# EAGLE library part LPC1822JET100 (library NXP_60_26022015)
32-bit ARM Cortex-M3 MCU; up to 1 MB flash and 136 kB SRAM; Ethernet, two High-speed USB, LCD, EMC The LPC185x/3x/2x/1x are ARM Cortex-M3 based microcontrollers for embedded applications. The ARM Cortex-M3 is a next generation core that offers system enhancements such as low power consumption, enhanced debug features, and a high level of support block integration. The LPC185x/3x/2x/1x operate at CPU frequencies of up to 180 MHz. The ARM Cortex-M3 CPU incorporates a 3-stage pipeline and uses a Harvard architecture with separate local instruction and data buses as well as a third bus for peripherals. The ARM Cortex-M3 CPU also includes an internal prefetch unit that supports speculative branching. The LPC185x/3x/2x/1x include up to 1 MB of flash and 136 kB of on-chip SRAM, 16 kB of EEPROM memory, a quad SPI Flash Interface (SPIFI), a State Configurable Timer (SCT) subsystem, two High-speed USB controllers, Ethernet, LCD, an external memory controller, and multiple digital and analog peripherals. AAL Eindhoven MK
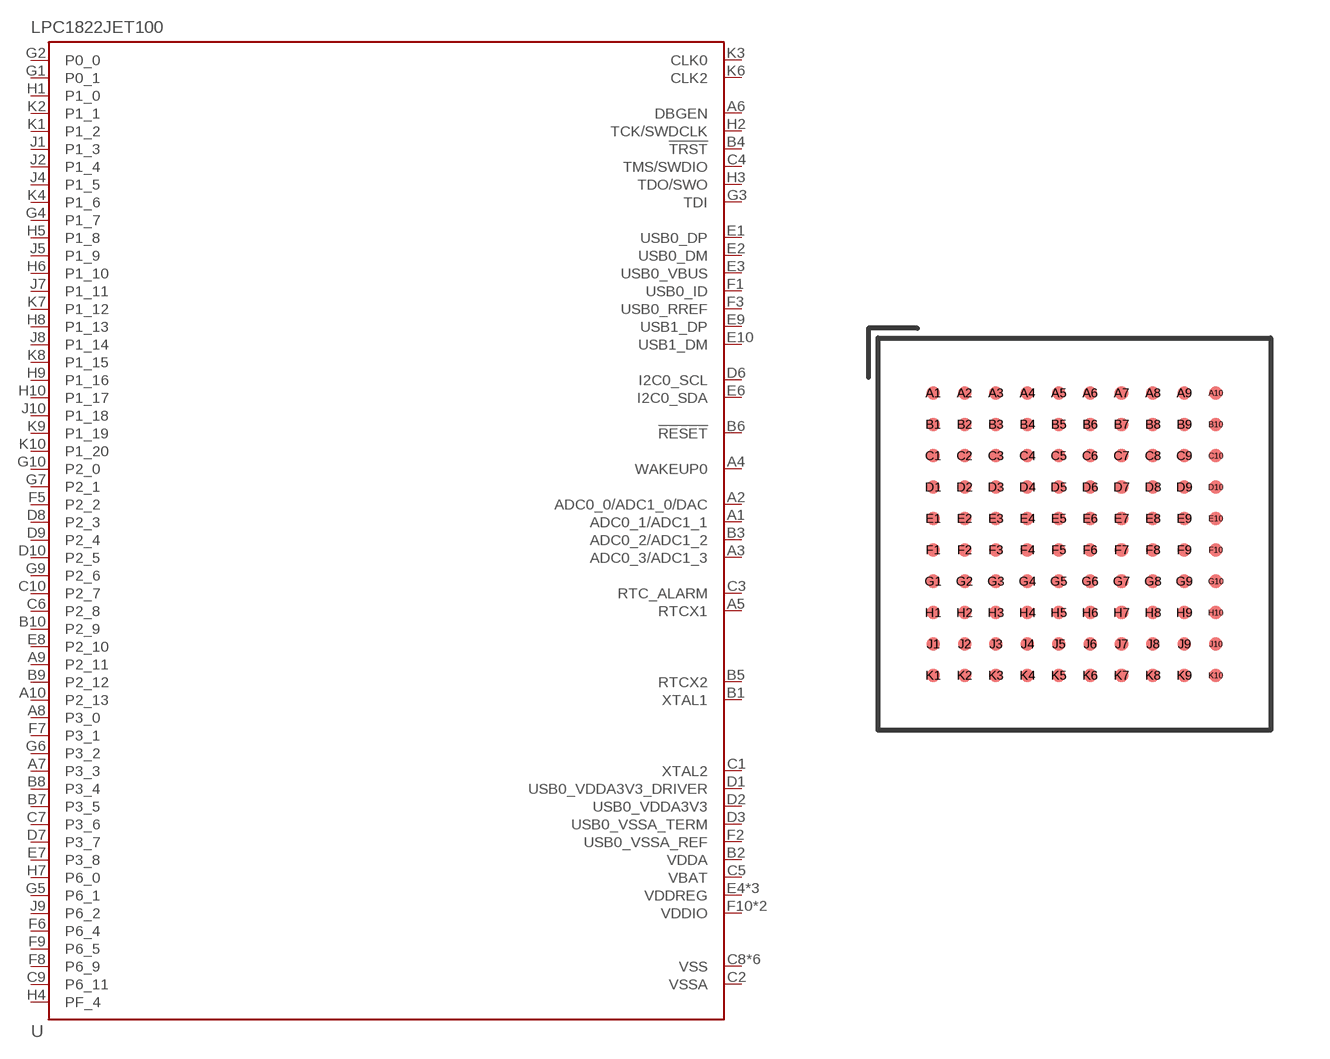
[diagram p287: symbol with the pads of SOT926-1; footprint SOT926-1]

Designator prefix U

## LPC1822JET100 (ADC: 4; ETHERNET: yes; FLASH: 512kB (1 bank); GPIO: 49; LCD: no; PWM: no; QEI: no; SRAM: 104kB; TEMPERATURE_RANGE: -40 °C to +105 °C; USB0: Host/OTG; USB1: No)  [SOT926-1]
A1  ADC0_1/ADC1_1
A2  ADC0_0/ADC1_0/DAC
A3  ADC0_3/ADC1_3
A4  WAKEUP0
A5  RTCX1
A6  DBGEN
A7  P3_3
A8  P3_0
A9  P2_11
A10  P2_13
B1  XTAL1
B2  VDDA
B3  ADC0_2/ADC1_2
B4  !TRST!
B5  RTCX2
B6  !RESET!
B7  P3_5
B8  P3_4
B9  P2_12
B10  P2_9
C1  XTAL2
C2  VSSA
C3  RTC_ALARM
C4  TMS/SWDIO
C5  VBAT
C6  P2_8
C7  P3_6
C8  VSS
C9  P6_11
C10  P2_7
D1  USB0_VDDA3V3_DRIVER
D2  USB0_VDDA3V3
D3  USB0_VSSA_TERM
D4  VSS
D5  VSS
D6  I2C0_SCL
D7  P3_7
D8  P2_3
D9  P2_4
D10  P2_5
E1  USB0_DP
E2  USB0_DM
E3  USB0_VBUS
E4  VDDREG
E5  VDDREG
E6  I2C0_SDA
E7  P3_8
E8  P2_10
E9  USB1_DP
E10  USB1_DM
F1  USB0_ID
F2  USB0_VSSA_REF
F3  USB0_RREF
F4  VDDREG
F5  P2_2
F6  P6_4
F7  P3_1
F8  P6_9
F9  P6_5
F10  VDDIO
G1  P0_1
G2  P0_0
G3  TDI
G4  P1_7
G5  P6_1
G6  P3_2
G7  P2_1
G8  VSS
G9  P2_6
G10  P2_0
H1  P1_0
H2  TCK/SWDCLK
H3  TDO/SWO
H4  PF_4
H5  P1_8
H6  P1_10
H7  P6_0
H8  P1_13
H9  P1_16
H10  P1_17
J1  P1_3
J2  P1_4
J3  VSS
J4  P1_5
J5  P1_9
J6  VSS
J7  P1_11
J8  P1_14
J9  P6_2
J10  P1_18
K1  P1_2
K2  P1_1
K3  CLK0
K4  P1_6
K5  VDDIO
K6  CLK2
K7  P1_12
K8  P1_15
K9  P1_19
K10  P1_20

## Footprint SOT926-1 (pad centres in mm)
SOT926-1 TFBGA100: plastic thin fine-pitch ball grid array package; 100 balls; body 9 x 9 x 0.7 mm JEDEC: -- IEC: --
smd 0.35 x 0.35: A1 -3.6,3.6; A2 -2.8,3.6; A3 -2,3.6; A4 -1.2,3.6; A5 -0.4,3.6; A6 0.4,3.6; A7 1.2,3.6; A8 2,3.6; A9 2.8,3.6; A10 3.6,3.6; B1 -3.6,2.8; B2 -2.8,2.8; B3 -2,2.8; B4 -1.2,2.8; B5 -0.4,2.8; B6 0.4,2.8; B7 1.2,2.8; B8 2,2.8; B9 2.8,2.8; B10 3.6,2.8; C1 -3.6,2; C2 -2.8,2; C3 -2,2; C4 -1.2,2; C5 -0.4,2; C6 0.4,2; C7 1.2,2; C8 2,2; C9 2.8,2; C10 3.6,2; D1 -3.6,1.2; D2 -2.8,1.2; D3 -2,1.2; D4 -1.2,1.2; D5 -0.4,1.2; D6 0.4,1.2; D7 1.2,1.2; D8 2,1.2; D9 2.8,1.2; D10 3.6,1.2; E1 -3.6,0.4; E2 -2.8,0.4; E3 -2,0.4; E4 -1.2,0.4; E5 -0.4,0.4; E6 0.4,0.4; E7 1.2,0.4; E8 2,0.4; E9 2.8,0.4; E10 3.6,0.4; F1 -3.6,-0.4; F2 -2.8,-0.4; F3 -2,-0.4; F4 -1.2,-0.4; F5 -0.4,-0.4; F6 0.4,-0.4; F7 1.2,-0.4; F8 2,-0.4; F9 2.8,-0.4; F10 3.6,-0.4; G1 -3.6,-1.2; G2 -2.8,-1.2; G3 -2,-1.2; G4 -1.2,-1.2; G5 -0.4,-1.2; G6 0.4,-1.2; G7 1.2,-1.2; G8 2,-1.2; G9 2.8,-1.2; G10 3.6,-1.2; H1 -3.6,-2; H2 -2.8,-2; H3 -2,-2; H4 -1.2,-2; H5 -0.4,-2; H6 0.4,-2; H7 1.2,-2; H8 2,-2; H9 2.8,-2; H10 3.6,-2; J1 -3.6,-2.8; J2 -2.8,-2.8; J3 -2,-2.8; J4 -1.2,-2.8; J5 -0.4,-2.8; J6 0.4,-2.8; J7 1.2,-2.8; J8 2,-2.8; J9 2.8,-2.8; J10 3.6,-2.8; K1 -3.6,-3.6; K2 -2.8,-3.6; K3 -2,-3.6; K4 -1.2,-3.6; K5 -0.4,-3.6; K6 0.4,-3.6; K7 1.2,-3.6; K8 2,-3.6; K9 2.8,-3.6; K10 3.6,-3.6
